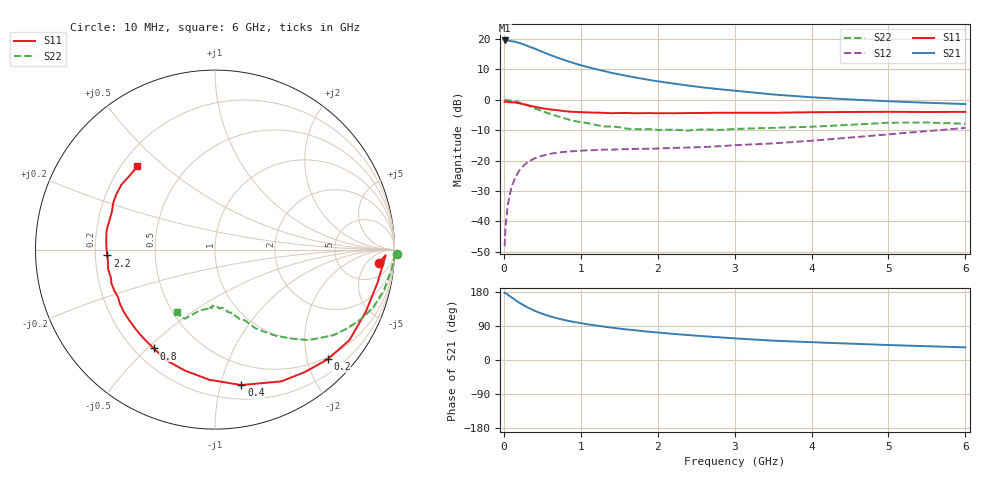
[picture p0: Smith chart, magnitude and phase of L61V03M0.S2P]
!  INFINEON TECHNOLOGIES Small Signal Semiconductors
! BFR380L3 , Si-NPN RF-Transistor in TSLP-3-1
!  Vce=1 V,  Ic=3 mA
! Common Emitter S-Parameters:  07. March 2005
#  GHz  S  MA  R  50
! f  S11  S21  S12  S22
! GHz  Mag  Ang  Mag  Ang  Mag  Ang  Mag  Ang
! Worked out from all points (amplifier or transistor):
!   36 points, 10 MHz to 6 GHz, reference 50 ohm
!   highest |S21| = 19.5 dB at 10 MHz (marker M1)
!   |S21| within 3 dB of that: start of sweep to 429.7 MHz
!   unconditionally stable (mu >= 1): 2.571 GHz to 4.855 GHz
!   at 250 MHz: K = 0.12, MSG = 20.1 dB, |S12| = -21.9 dB
!   at 1.4 GHz: K = 0.66, MSG = 12.6 dB, |S12| = -16.4 dB
!   at 6 GHz: K = 0.95, MSG = 3.9 dB, |S12| = -9.2 dB
!   S11 on the Smith chart (normalised r, x): 10 MHz: 12, -11; 200 MHz: 0.45, -2.38; 400 MHz: 0.32, -1.16; 800 MHz: 0.28, -0.52; 2.2 GHz: 0.25, -0.03; 6 GHz: 0.26, +0.41
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0.01  0.9148 -4.7  9.482 176.9  0.0039 81.0  1.013 -1.4
0.02  0.9513 -1.9  9.466 177.4  0.0072 87.5  0.9991 -2.9
0.05  0.924 -11.6  9.434 172.6  0.0185 84.4  0.9886 -6.8
0.1  0.9089 -22.4  9.208 165.5  0.0371 77.6  0.9679 -13.5
0.15  0.9032 -34.0  9.003 158.2  0.0534 71.9  0.9392 -20.0
0.2  0.8758 -44.3  8.629 151.4  0.0682 66.9  0.9017 -25.4
0.25  0.8467 -53.6  8.229 145.5  0.0807 61.7  0.8555 -31.0
0.3  0.8224 -63.2  7.778 139.6  0.0921 57.4  0.8151 -35.8
0.4  0.7688 -79.0  6.955 129.8  0.1091 50.3  0.7253 -44.1
0.5  0.7262 -92.4  6.172 122.0  0.1204 45.0  0.649 -49.7
0.6  0.6942 -104.1  5.483 115.1  0.1289 40.9  0.5877 -54.8
0.8  0.6478 -121.8  4.457 104.9  0.1395 36.0  0.4906 -63.0
0.9  0.6338 -129.5  4.048 100.8  0.1425 34.3  0.4508 -65.4
1.1  0.6192 -140.6  3.433 93.8  0.1476 32.6  0.4105 -70.4
1.5  0.6059 -158.0  2.623 82.9  0.153 32.3  0.3538 -78.4
1.9  0.605 -169.8  2.113 74.4  0.1565 34.0  0.3288 -85.8
2.2  0.601 -176.9  1.857 69.0  0.1615 36.1  0.3225 -88.1
2.8  0.6121 171.2  1.497 59.9  0.172 42.1  0.3188 -96.6
3.5  0.6113 160.3  1.224 51.0  0.1918 48.0  0.3457 -102.7
4.5  0.6302 150.6  1.014 43.2  0.239 56.0  0.3871 -109.6
5.5  0.6294 139.5  0.894 36.4  0.3053 58.6  0.4224 -116.8
6  0.6342 133.0  0.852 33.4  0.3451 58.2  0.4039 -121.3
